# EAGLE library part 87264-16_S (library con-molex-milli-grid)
RECEPTACAL
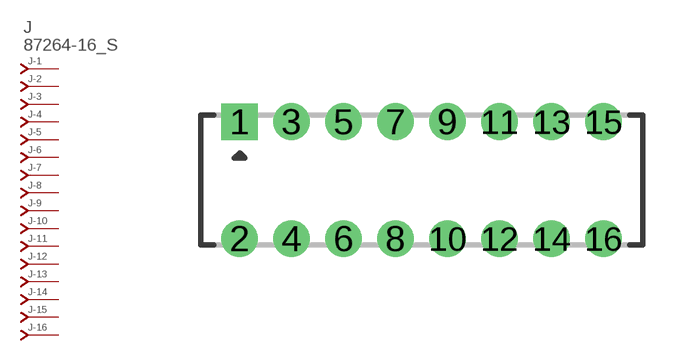
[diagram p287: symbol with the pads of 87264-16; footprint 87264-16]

Designator prefix J; gates -1=J-NV -2=J-N -3=J-N -4=J-N -5=J-N -6=J-N -7=J-N -8=J-N -9=J-N -10=J-N -11=J-N -12=J-N -13=J-N -14=J-N -15=J-N -16=J-N

## 87264-16_S  [87264-16]
1  -1:J  pas
2  -2:J  pas
3  -3:J  pas
4  -4:J  pas
5  -5:J  pas
6  -6:J  pas
7  -7:J  pas
8  -8:J  pas
9  -9:J  pas
10  -10:J  pas
11  -11:J  pas
12  -12:J  pas
13  -13:J  pas
14  -14:J  pas
15  -15:J  pas
16  -16:J  pas

## Footprint 87264-16 (pad centres in mm)
RECEPTACAL Dual Row, Side Entry
drill 0.914 square: 1 -7,2.25
drill 0.914: 2 -7,-2.25; 3 -5,2.25; 4 -5,-2.25; 5 -3,2.25; 6 -3,-2.25; 7 -1,2.25; 8 -1,-2.25; 9 1,2.25; 10 1,-2.25; 11 3,2.25; 12 3,-2.25; 13 5,2.25; 14 5,-2.25; 15 7,2.25; 16 7,-2.25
